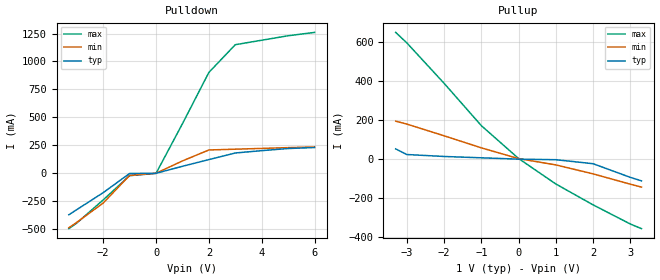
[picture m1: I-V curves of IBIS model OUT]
[IBIS Ver]   2.1
[File Name]   bug19.ibs
[File Rev]   2.0
[Component]   A
[Manufacturer]  anyone
[Package]
|   typ   min   max
R_pkg   1.0   2.0   3.0
L_pkg   1.0n   2.0n   3.0n
C_pkg   1.0p   2.0p   3.0p
[Pin]   signal_name   model_name   R_pin   L_pin   C_pin
18   1Y1   OUT
19   1Y2   OUT
[Diff Pin] inv_pin  vdiff tdelay_typ   tdelay_min   tdelay_max
18   19   .1   2n   3n   4n
| Models and submodels in the file (1): OUT (3-state)
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[Model]   OUT
Model_type   3-state
|   typ   min   max
C_comp   1.0p   2.0p   3.0p
[Voltage range]   1.0   2.0   3.0
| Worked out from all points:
|   slope of the pulldown table from 0 to 0.15 V, typ, clamps not added: 16 ohm
|   slope of the pullup table from 0 to 0.15 V, typ, clamps not added: 345 ohm
[Pullup]
|Voltage   I(typ)   I(min)   I(max)
-3.3V     53mA       195mA      650mA
-3V       24mA       180mA      596mA
-2V       14mA       120mA      389mA
-1V       7.2mA      58.2mA     172mA
0V        300uA      3mA        3.6mA
1V        -2.6mA     -29.2mA    -127mA
2V        -23mA      -75.1mA    -234mA
3V        -93mA      -128mA     -332mA
3.3V      -111mA     -143mA     -356mA
[Pulldown]
|Voltage   I(typ)   I(min)   I(max)
-3.3V     -372mA     -488mA     -496mA
-3V       -326mA     -440mA     -446mA
-2V       -174mA     -267mA     -239mA
-1V       -2.2mA     -19.6mA    -21.8mA
0V        -670uA     -460uA     -1.43mA
1V        62mA       110mA      443mA
2V        122mA      208mA      902mA
3V        181mA      215mA      1.15A
4V        202mA      222mA      1.19A
5V        221mA      229mA      1.23A
6V        230mA      235mA      1.26A
[Ramp]
|Variable   typ   min   max
dV/dt_r   1.000/1.000n   2.000/1.000n   3.000/1.000n
dV/dt_f   1.000/1.000n   2.000/1.000n   3.000/1.000n
